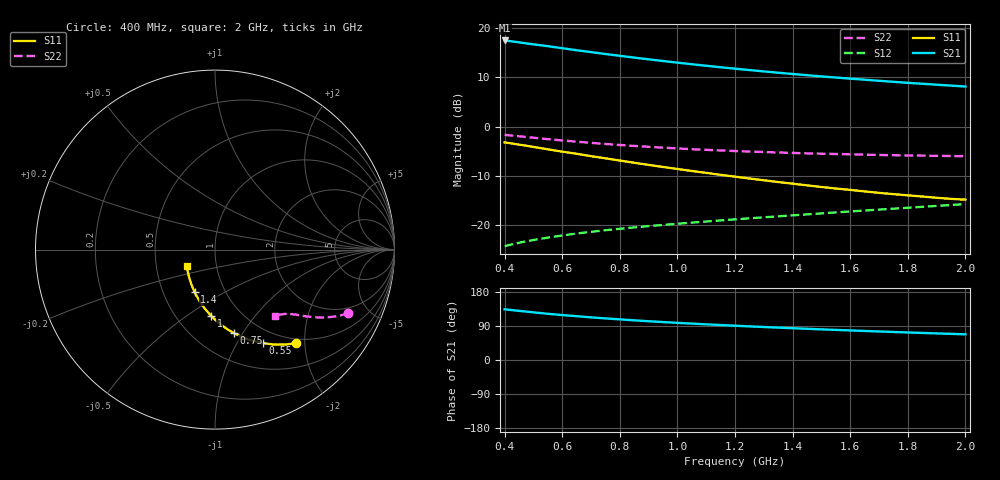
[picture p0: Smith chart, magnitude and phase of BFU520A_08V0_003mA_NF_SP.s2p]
! Filename:  P:\Prog\Test\Noise\ATS_data\Testdata_Net\06 Compressed Noise after Statistics\BFU520A_APG2013_30_A05_08p0V_003mA_NF_CM01_D.sf
! Date/Time: Wed 24/Apr/2013 20:06:19
! BFU520A_APG2013_30_A05_08p0V_1to20mA_NF_CM01_Bias3_R.sf
! Noise Parameter Data File
! BFU520A_APG2013_30_A05_08p0V_1to20mA_NF_CM01
! Date/time: Thu Apr 11 09:33:54 2013
! VAR V_out= 8.001000
! VAR I_out= 2.995000
! VAR V_in= 0.815200
! VAR I_in= 0.031605
! Device data file deembeded for feedlines and parallel
! Original file: \06 Compressed Noise after Statistics\BFU520A_APG2013_30_A05_08p0V_003mA_NF_CM01_R.sf
! Feed-files: PR017V01_150413_Feed1.s2p, PR017V01_150413_Feed2.s2p
! Parallel-file: PR017V01_150413_Par.s2p
# MHz S MA R 50
!  Freq-MHz  S11-mag  S11-arg  S21-mag  S21-arg  S12-mag  S12-arg  S22-mag  S22-arg
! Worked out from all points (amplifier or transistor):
!   37 points, 400 MHz to 2 GHz, reference 50 ohm
!   highest |S21| = 17.5 dB at 400 MHz (marker M1)
!   |S21| within 3 dB of that: start of sweep to 783.3 MHz
!   unconditionally stable (mu >= 1): 1.9 GHz to end of sweep
!   at 500 MHz: K = 0.46, MSG = 19.9 dB, |S12| = -23.1 dB
!   at 1.1 GHz: K = 0.82, MSG = 15.8 dB, |S12| = -19.3 dB
!   at 2 GHz: K = 1.01, MAG = 11.4 dB, |S12| = -15.8 dB
!   lowest NFmin = 0.56 dB at 420 MHz
!   S11 on the Smith chart (normalised r, x): 400 MHz: 0.92, -1.82; 550 MHz: 0.81, -1.29; 750 MHz: 0.76, -0.91; 1 GHz: 0.73, -0.63; 1.4 GHz: 0.72, -0.37; 2 GHz: 0.72, -0.13
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400  0.69 -49.0  7.482 133.9  0.06088 65.1  0.8224 -25.4
420  0.6757 -51.0  7.356 132.1  0.06296 64.3  0.8113 -26.2
460  0.6479 -54.8  7.091 128.8  0.06683 63.1  0.7905 -27.6
500  0.6205 -58.4  6.836 125.7  0.07038 62.0  0.7691 -28.9
550  0.5867 -62.8  6.545 122.0  0.07434 60.8  0.7436 -30.4
600  0.5555 -66.8  6.242 118.6  0.07818 59.9  0.7216 -31.6
650  0.5283 -70.4  5.953 115.6  0.08181 59.1  0.7014 -32.7
700  0.5 -74.1  5.701 112.5  0.0851 58.6  0.6823 -33.6
750  0.4752 -77.4  5.447 109.8  0.08833 58.1  0.6649 -34.5
800  0.4512 -80.9  5.224 107.2  0.09142 57.8  0.6491 -35.2
850  0.4283 -84.1  5.011 104.7  0.0944 57.5  0.6348 -36.0
900  0.4075 -87.3  4.813 102.3  0.09734 57.4  0.622 -36.6
950  0.3879 -90.2  4.627 100.1  0.1001 57.4  0.6093 -37.2
1000  0.3706 -93.1  4.452 98.0  0.1028 57.4  0.5989 -37.8
1100  0.3381 -99.0  4.139 94.1  0.1084 57.5  0.5793 -38.7
1200  0.3095 -104.6  3.867 90.5  0.1139 57.8  0.5634 -39.8
1300  0.2844 -109.9  3.628 87.0  0.1195 58.1  0.5506 -40.8
1400  0.2627 -115.6  3.415 83.9  0.1252 58.5  0.5392 -41.7
1500  0.243 -121.3  3.228 80.9  0.131 59.0  0.5291 -42.6
1650  0.219 -129.7  2.988 76.6  0.1401 59.6  0.5179 -44.2
1750  0.2056 -135.6  2.843 74.0  0.1463 60.0  0.5106 -45.2
2000  0.1807 -150.4  2.549 67.8  0.1629 60.9  0.4992 -48.0
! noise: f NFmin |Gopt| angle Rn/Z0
400  0.6014  0.3789  15.42  0.1703
460  0.5833  0.3675  20.77  0.1631
600  0.6864  0.36  21.46  0.1805
800  0.6597  0.3306  39.24  0.1427
1000  0.6865  0.3332  49.56  0.1358
1200  0.7283  0.3175  58.44  0.1322
1400  0.7534  0.2948  72.45  0.1194
1600  0.777  0.27  85.85  0.0999
1800  0.7472  0.2286  102.4  0.0903
2000  0.7803  0.2502  112.2  0.083
